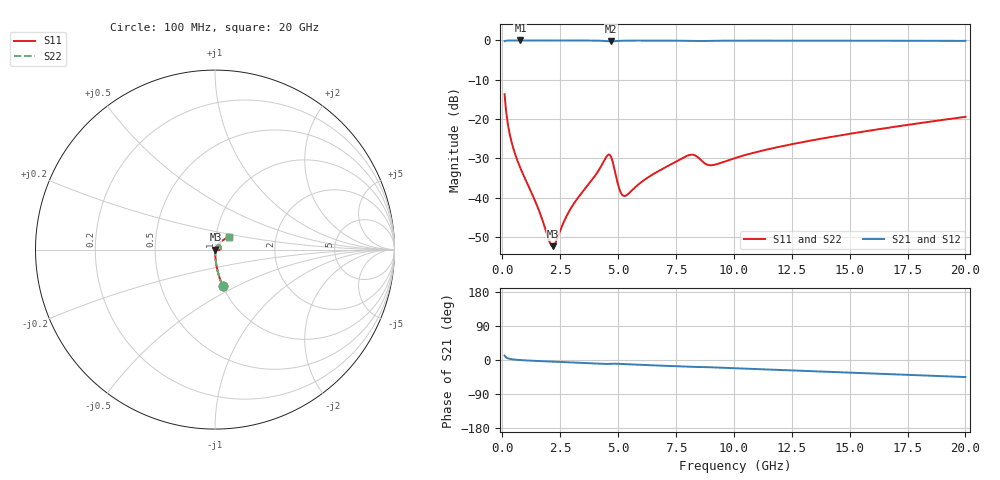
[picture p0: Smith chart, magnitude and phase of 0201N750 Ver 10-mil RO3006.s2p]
# GHz S MA R 50
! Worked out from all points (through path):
!   1601 points, 100 MHz to 20 GHz, reference 50 ohm
!   highest |S21| = -0.01 dB at 784.1 MHz (marker M1); lowest = -0.3 dB at 4.677 GHz (marker M2)
!   group delay of S21, straight-line fit = 6.38 ps
!   lowest |S11| = -52.3 dB at 2.177 GHz (marker M3), VSWR 1.00, Z = 50.2 - j0.0332 ohm
!   |S11| at or under -10 dB: start of sweep to end of sweep
!   |S22| runs from -52.3 to -13.7 dB; largest |S21 - S12| = 0
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0.1  0.2067 -78.0  0.9775 11.7  0.9775 11.7  0.2067 -78.0
0.2616875  0.07953 -85.3  0.9959 4.0  0.9959 4.0  0.07953 -85.3
0.373625  0.055 -86.5  0.9974 2.4  0.9974 2.4  0.055 -86.5
0.7840625  0.02372 -86.8  0.9983 -0.2  0.9983 -0.2  0.02372 -86.8
1.530312  0.007542 -77.4  0.9979 -2.6  0.9979 -2.6  0.007542 -77.4
2.04025  0.002744 -36.2  0.9976 -4.0  0.9976 -4.0  0.002744 -36.2
2.177062  0.002414 -7.9  0.9975 -4.4  0.9975 -4.4  0.002414 -7.9
2.313875  0.002732 19.2  0.9974 -4.7  0.9974 -4.7  0.002732 19.2
2.861125  0.006503 57.5  0.997 -6.1  0.997 -6.1  0.006503 57.5
3.420812  0.01139 64.5  0.9963 -7.5  0.9963 -7.5  0.01139 64.5
4.03025  0.01939 63.2  0.9938 -9.1  0.9938 -9.1  0.01939 63.2
4.502875  0.0333 40.8  0.9787 -10.5  0.9787 -10.5  0.0333 40.8
4.677  0.03393 14.0  0.9688 -10.1  0.9688 -10.1  0.03393 14.0
5.062563  0.0127 1.1  0.9874 -10.3  0.9874 -10.3  0.0127 1.1
5.249125  0.01051 22.4  0.9911 -10.8  0.9911 -10.8  0.01051 22.4
6.741625  0.02172 60.6  0.9941 -14.7  0.9941 -14.7  0.02172 60.6
8.122188  0.03507 46.8  0.9844 -18.0  0.9844 -18.0  0.03507 46.8
8.967937  0.02586 42.5  0.9872 -19.1  0.9872 -19.1  0.02586 42.5
10.05  0.03186 55.5  0.9922 -21.7  0.9922 -21.7  0.03186 55.5
13.37081  0.05352 53.7  0.9919 -29.4  0.9919 -29.4  0.05352 53.7
16.69162  0.07763 47.7  0.9896 -37.2  0.9896 -37.2  0.07763 47.7
20  0.1066 40.8  0.9861 -45.0  0.9861 -45.0  0.1066 40.8
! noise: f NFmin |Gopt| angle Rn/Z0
0.1  0.000592  0.9276  0.2346  0.001815
2.301  0.004735  0.8052  4.608  0.005043
4.515  0.01969  0.9033  9.022  0.04435
6.729  0.01208  0.7809  13.39  0.01115
8.943  0.02096  0.8286  17.77  0.02514
11.14  0.01661  0.7446  22  0.0126
13.36  0.01823  0.7259  26.22  0.01255
15.57  0.02022  0.7161  30.38  0.01313
17.79  0.02228  0.7095  34.48  0.01381
20  0.02436  0.7051  38.5  0.0145
